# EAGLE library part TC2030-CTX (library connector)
Tag Connect footprint for ARM JTAG. 10 pin ARM Cortex Debug Connector.
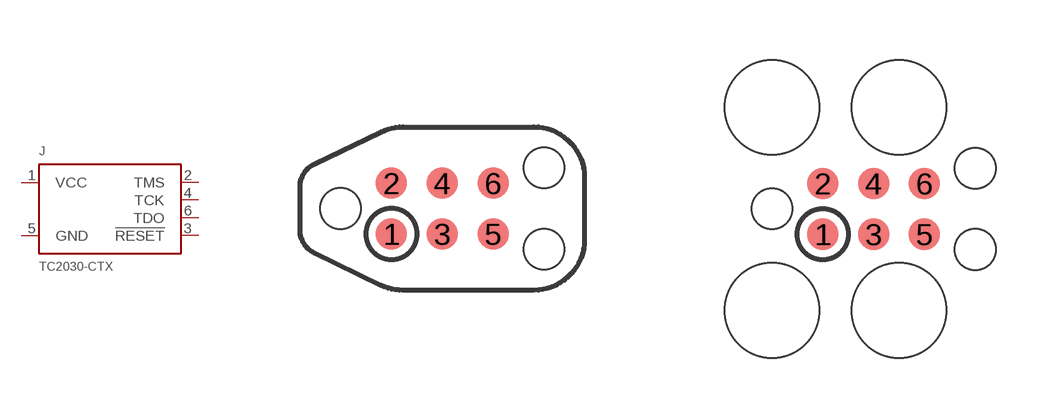
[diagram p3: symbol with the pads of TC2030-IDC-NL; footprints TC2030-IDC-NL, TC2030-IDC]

Designator prefix J

## TC2030-CTX-NL  [TC2030-IDC-NL]
1  VCC
2  TMS
3  !RESET
4  TCK
5  GND
6  TDO

## TC2030-CTX  [TC2030-IDC]
Pads as for TC2030-IDC-NL

## Footprint TC2030-IDC-NL (pad centres in mm)
The TC2030-IDC-NL is our "No Legs" 6-pin Plug-of-Nails Cable
smd 0.787 x 0.787: 1 -1.27,-0.635; 2 -1.27,0.635; 3 0,-0.635; 4 0,0.635; 5 1.27,-0.635; 6 1.27,0.635
hole 1.016 at -2.54,0
hole 1.016 at 2.54,1.016
hole 1.016 at 2.54,-1.016

## Footprint TC2030-IDC (pad centres in mm)
Tag Connect TC2030-IDC
smd 0.787 x 0.787: 1 -1.27,-0.635; 2 -1.27,0.635; 3 0,-0.635; 4 0,0.635; 5 1.27,-0.635; 6 1.27,0.635
hole 2.375 at -2.54,2.54
hole 2.375 at 0.635,2.54
hole 2.375 at 0.635,-2.54
hole 2.375 at -2.54,-2.54
hole 1.016 at -2.54,0
hole 1.016 at 2.54,1.016
hole 1.016 at 2.54,-1.016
